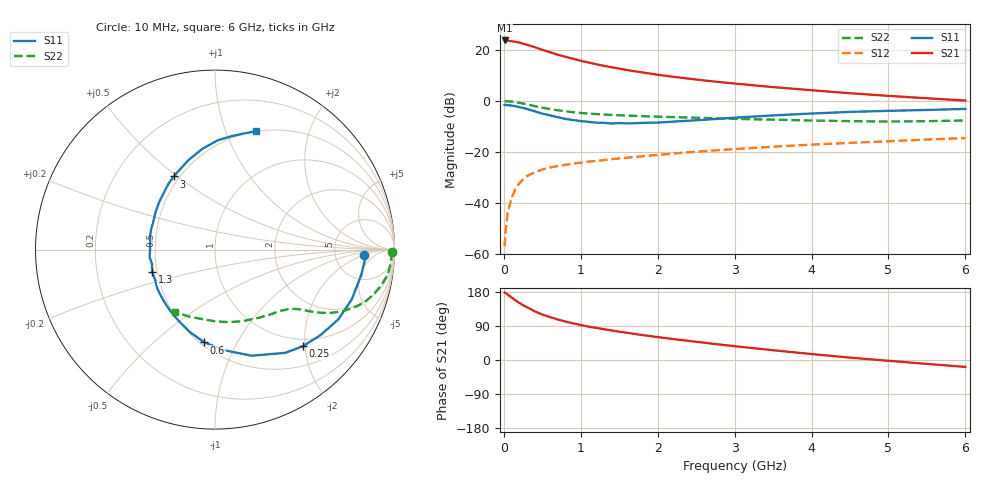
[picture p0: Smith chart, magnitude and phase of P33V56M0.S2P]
! SIEMENS Small Signal Semiconductors
! BFP181
! Si NPN RF Bipolar Junction Transistor in SOT143
! VCE = 3.5 V  IC = 6 mA
! Common Emitter S-Parameters:  March  1996
# GHz  S  MA  R  50
!  f  S11  S21  S12  S22
! GHz  MAG  ANG  MAG  ANG  MAG  ANG  MAG  ANG
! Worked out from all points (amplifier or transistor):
!   36 points, 10 MHz to 6 GHz, reference 50 ohm
!   highest |S21| = 23.8 dB at 10 MHz (marker M1)
!   |S21| within 3 dB of that: start of sweep to 436 MHz
!   unconditionally stable (mu >= 1): 1.568 GHz to end of sweep
!   at 250 MHz: K = 0.24, MSG = 26.7 dB, |S12| = -30.9 dB
!   at 1.4 GHz: K = 0.96, MSG = 18.1 dB, |S12| = -22.9 dB
!   at 6 GHz: K = 1.04, MAG = 6.2 dB, |S12| = -14.6 dB
!   S11 on the Smith chart (normalised r, x): 10 MHz: 11, -2; 250 MHz: 0.86, -1.96; 600 MHz: 0.52, -0.74; 1.3 GHz: 0.47, -0.14; 3 GHz: 0.46, +0.49; 6 GHz: 0.50, +1.28
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0.01  0.8323 -2.1  15.43 178.3  0.0014 79.8  0.9887 -0.8
0.05  0.8276 -9.7  15.34 172.4  0.0064 88.7  0.983 -4.3
0.1  0.8109 -20.0  14.91 165.0  0.0123 79.1  0.9718 -8.4
0.15  0.7892 -29.6  14.52 157.7  0.0185 73.4  0.9468 -12.2
0.2  0.7565 -39.1  14.07 150.9  0.0241 70.8  0.9187 -15.7
0.25  0.7277 -47.7  13.32 144.6  0.0286 65.9  0.888 -18.9
0.3  0.6956 -55.8  12.7 139.5  0.0333 62.8  0.8565 -21.4
0.4  0.6253 -71.0  11.42 128.6  0.0396 56.8  0.7934 -25.6
0.5  0.5638 -84.4  10.1 120.0  0.0449 52.1  0.7366 -28.6
0.6  0.5206 -96.6  9.085 113.1  0.0492 49.5  0.6914 -30.6
0.7  0.4791 -107.2  8.093 107.0  0.0527 47.3  0.6549 -32.2
0.8  0.4444 -117.6  7.385 101.5  0.0556 45.7  0.6256 -33.2
0.9  0.4201 -127.4  6.739 96.7  0.0587 44.7  0.6005 -34.2
1.1  0.3888 -145.5  5.705 88.1  0.0642 43.3  0.564 -36.0
1.3  0.3715 -160.2  4.894 81.3  0.0689 42.6  0.5401 -37.7
1.7  0.3645 172.8  3.836 68.7  0.0793 41.4  0.5085 -41.7
2.2  0.3919 147.7  2.986 55.3  0.0924 39.8  0.4813 -47.6
3  0.4682 119.5  2.199 36.4  0.1132 36.0  0.4446 -59.5
3.5  0.5193 106.7  1.87 25.8  0.1263 33.1  0.4283 -68.4
4.5  0.6089 88.6  1.417 6.3  0.1499 26.6  0.4005 -89.3
5.5  0.6652 76.3  1.127 -10.3  0.1744 20.4  0.4005 -111.6
6  0.6972 71.0  1.018 -18.3  0.1864 16.6  0.4122 -123.0
